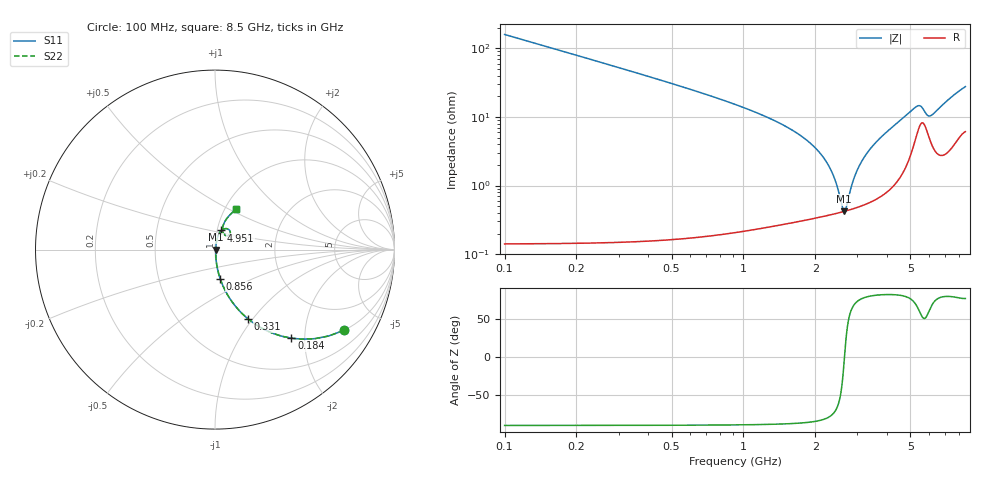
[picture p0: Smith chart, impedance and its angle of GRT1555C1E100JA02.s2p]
!Murata Part Number: GRT1555C1E100JA02
!These Parameters are Measured in Series Mode Connection
!Data Generated on Jun 19, 2026
!  o--ll--o
!Port1  Port2
!  o------o
!Operation Temp=25[degC], DC Bias Voltage=0[V]
!Freq. Start=100[MHz] Stop=9[GHz] 401[Steps]
# Hz S RI R 50
!Freq.(Hz) S11(Real) S11(Imag) S21(Real) S21(Imag) S12(Real) S12(Imag) S22(Real) S22(Imag)
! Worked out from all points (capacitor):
!   401 points, 100 MHz to 8.5 GHz, reference 50 ohm
!   read as one part in series: C = 10 pF near 142 MHz
!   lowest |Z| = 421 mohm at 2.641 GHz (marker M1)
!   series resonance near 2.649 GHz, so ESL is about 360 pH
!   S11 on the Smith chart (normalised r, x): 100 MHz: 1.00, -3.18; 184 MHz: 1.00, -1.72; 331 MHz: 1.00, -0.95; 856 MHz: 1.00, -0.33; 4.951 GHz: 1.05, +0.23; 8.5 GHz: 1.12, +0.54
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1e8  0.7162 -0.4504  0.2838 0.4504  0.2838 0.4504  0.7162 -0.4504
1.84e8  0.4258 -0.4936  0.5742 0.4936  0.5742 0.4936  0.4258 -0.4936
3.31e8  0.1839 -0.3858  0.8161 0.3858  0.8161 0.3858  0.1839 -0.3858
5.2e8  0.0811 -0.2702  0.9189 0.2702  0.9189 0.2702  0.0811 -0.2702
8.56e8  0.029 -0.1619  0.971 0.1619  0.971 0.1619  0.029 -0.1619
1.507e9  0.00792 -0.0716  0.9921 0.0716  0.9921 0.0716  0.00792 -0.0716
1.927e9  0.00482 -0.0396  0.9952 0.0396  0.9952 0.0396  0.00482 -0.0396
2.221e9  0.00409 -0.0219  0.9959 0.0219  0.9959 0.0219  0.00409 -0.0219
2.41e9  0.00399 -0.0118  0.996 0.0118  0.996 0.0118  0.00399 -0.0118
2.599e9  0.00412 -0.0024  0.9959 0.0024  0.9959 0.0024  0.00412 -0.0024
2.641e9  0.00418 -0.000378  0.9958 0.000378  0.9958 0.000378  0.00418 -0.000378
2.704e9  0.00428 0.00261  0.9957 -0.00261  0.9957 -0.00261  0.00428 0.00261
2.914e9  0.00477 0.0123  0.9952 -0.0123  0.9952 -0.0123  0.00477 0.0123
3.124e9  0.00549 0.0216  0.9945 -0.0216  0.9945 -0.0216  0.00549 0.0216
3.397e9  0.00679 0.0334  0.9932 -0.0334  0.9932 -0.0334  0.00679 0.0334
4.3e9  0.0157 0.0734  0.9843 -0.0734  0.9843 -0.0734  0.0157 0.0734
4.951e9  0.0358 0.1065  0.9642 -0.1065  0.9642 -0.1065  0.0358 0.1065
5.392e9  0.0742 0.1136  0.9258 -0.1136  0.9258 -0.1136  0.0742 0.1136
5.707e9  0.0799 0.0821  0.9201 -0.0821  0.9201 -0.0821  0.0799 0.0821
6.064e9  0.0502 0.0853  0.9498 -0.0853  0.9498 -0.0853  0.0502 0.0853
7.114e9  0.0542 0.1547  0.9458 -0.1547  0.9458 -0.1547  0.0542 0.1547
8.5e9  0.1147 0.225  0.8853 -0.225  0.8853 -0.225  0.1147 0.225
